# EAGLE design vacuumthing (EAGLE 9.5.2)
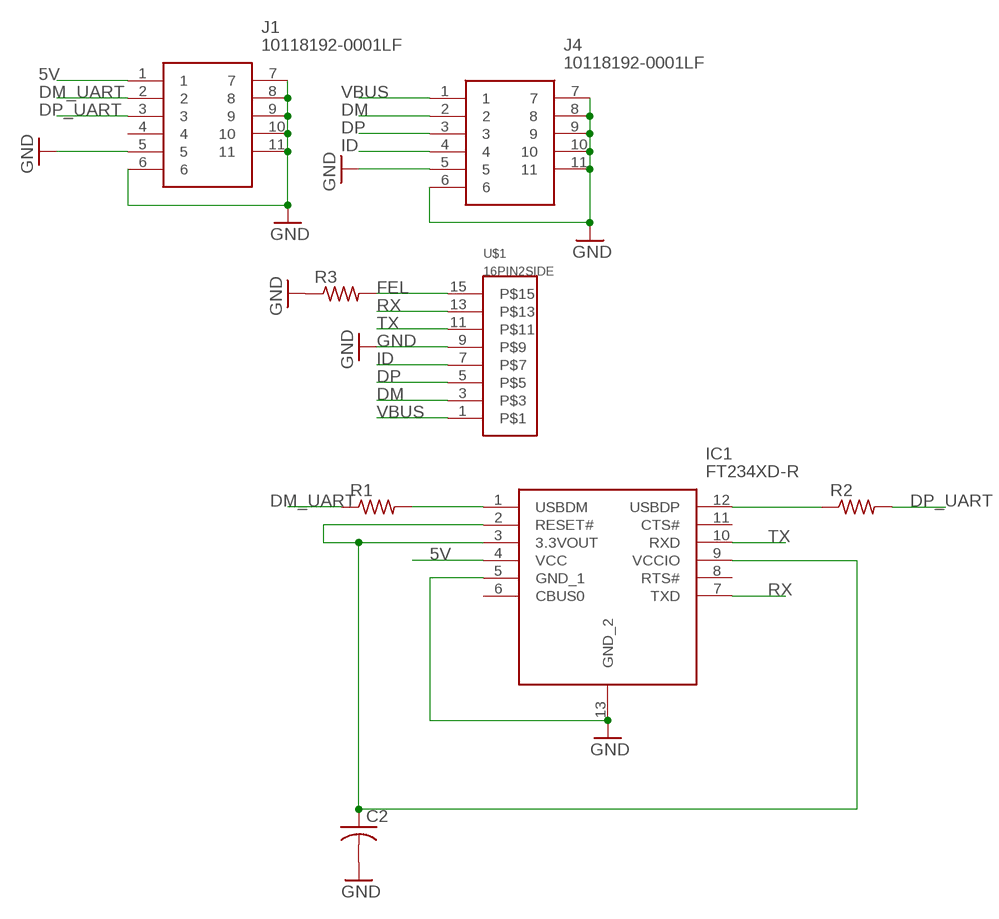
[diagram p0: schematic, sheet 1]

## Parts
C2  C-USC0402K  [C0402K]
IC1  FT234XD-R  [SON45P300X300X75-13N]
J1  10118192-0001LF  [101181920001LF]
J4  10118192-0001LF  [101181920001LF]
R1  R-US_R0402  [R0402]
R2  R-US_R0402  [R0402]
R3  R-US_R0603  [R0603]
U$1  16PIN2SIDE  [16PIN2SIDE]

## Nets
5V: IC1.4(VCC) J1.1
DM: J4.2 U$1.3
DM_UART: J1.2 R1.1
DP: J4.3 U$1.5
DP_UART: J1.3 R2.2
FEL: R3.2 U$1.15
GND: C2.2 IC1.5(GND_1) IC1.13(GND_2) J1.5 J1.6 J1.7 J1.8 J1.9 J1.10 J1.11 J4.5 J4.6 J4.7 J4.8 J4.9 J4.10 J4.11 R3.1 U$1.9
ID: J4.4 U$1.7
N$2: C2.1 IC1.2(RESET#) IC1.3(3.3VOUT) IC1.9(VCCIO)
N$4: IC1.1(USBDM) R1.2
N$7: IC1.12(USBDP) R2.1
RX: IC1.7(TXD) U$1.13
TX: IC1.10(RXD) U$1.11
VBUS: J4.1 U$1.1
Unconnected: IC1.6(CBUS0) IC1.8(RTS#) IC1.11(CTS#) J1.4

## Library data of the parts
C2 = rcl:C-US: CAPACITOR, American symbol; SPICEPREFIX: C
IC1 = SamacSys_Parts:FT234XD-R: USB/UART IC, w/USB Charge Detection FTDI Chip FT234XD-R, USB Controller, 3MBd, USB 1.1, USB 2.0, 5 V, 12-Pin DFN Source: Datasheet; ARROW_PART_NUMBER: FT234XD-R; ARROW_PRICE-STOCK: https://www.arrow.com/en/products/ft234xd-r/ftdi-chip; DESCRIPTION: USB/UART IC, w/USB Charge Detection FTDI Chip FT234XD-R, USB Controller, 3MBd, USB 1.1, USB 2.0, 5 V, 12-Pin DFN; HEIGHT: 0.75mm; MANUFACTURER_NAME: FTDI Chip; MANUFACTURER_PART_NUMBER: FT234XD-R; MOUSER_PART_NUMBER: 895-FT234XD-R; MOUSER_PRICE-STOCK: https://www.mouser.co.uk/ProductDetail/FTDI/FT234XD-R?qs=NVftvxkm2tjipk322Ah1HQ%3D%3D
J1 J4 = SamacSys_Parts:10118192-0001LF: USB Connectors 5P MICRO USB TYPE B RECEPTACLE Source: Datasheet; ARROW_PART_NUMBER: 10118192-0001LF; ARROW_PRICE-STOCK: https://www.arrow.com/en/products/10118192-0001lf/amphenol-fci; DESCRIPTION: USB Connectors 5P MICRO USB TYPE B RECEPTACLE; HEIGHT: 2.8mm; MANUFACTURER_NAME: Amphenol; MANUFACTURER_PART_NUMBER: 10118192-0001LF; MOUSER_PART_NUMBER: 649-10118192-0001LF; MOUSER_PRICE-STOCK: https://www.mouser.co.uk/ProductDetail/Amphenol-FCI/10118192-0001LF/?qs=Ywefl8B65e5bHFoQtIudZg%3D%3D
R1-R3 = rcl:R-US_: RESISTOR, American symbol; SPICEPREFIX: R
U$1 = 16pin2.0:16PIN2SIDE

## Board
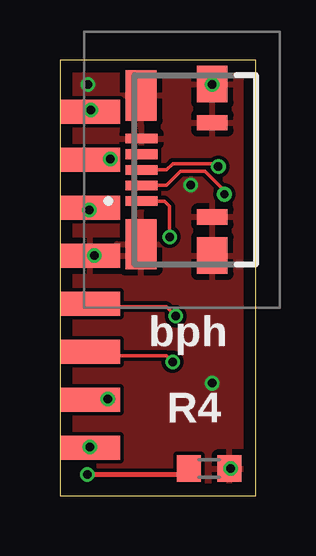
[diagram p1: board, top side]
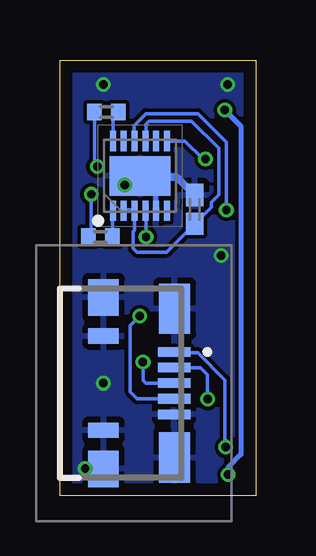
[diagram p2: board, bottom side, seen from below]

Size 8.17 x 18.16 mm. Coordinates in mm from the lower left corner, seen from the top.
Outline: 0,0 8.17,0 8.17,18.16 0,18.16 0,0
Copper layers (1*16): Top 0.035mm / dielectric 1.5mm / Bottom 0.035mm
Design rules "default *": minimum track width 6mil, minimum drill 0.35mm, track to track 6mil, track to pad 6mil, pad to pad 6mil, via to via 6mil, smd to smd 6mil, copper to edge 20mil, drill to drill 6mil, minimum pad ring 10mil, minimum via ring 0.13mm, stop-mask expansion 0mil, vias tented up to drill 30mil, thermal gap 10mil

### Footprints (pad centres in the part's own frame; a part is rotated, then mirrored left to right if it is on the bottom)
C0402K = smd 0.925 x 0.74: 1 -0.6,0; 2 0.6,0
SON45P300X300X75-13N = smd 0.85 x 0.25: 1 -1.45,1.125; 2 -1.45,0.675; 3 -1.45,0.225; 4 -1.45,-0.225; 5 -1.45,-0.675; 6 -1.45,-1.125; 7 1.45,-1.125; 8 1.45,-0.675; 9 1.45,-0.225; 10 1.45,0.225; 11 1.45,0.675; 12 1.45,1.125 | smd 1.65 x 2.55: 13 0,0
101181920001LF = smd 0.4 x 1.35: 1 -1.3,1.682; 2 -0.65,1.682; 3 0,1.682; 4 0.65,1.682; 5 1.3,1.682 | smd 2.1 x 1.295: 6 -3.1,1.702; 7 3.1,1.702 | smd 0.635 x 1.27: 8 -1.962,-1.27; 9 1.962,-1.27 | smd 1.524 x 1.27: 10 -3.571,-1.27; 11 3.571,-1.27
R0402 = smd 0.6 x 0.7: 1 -0.5,0; 2 0.5,0
R0603 = smd 1 x 1.1: 1 -0.85,0; 2 0.85,0
16PIN2SIDE = smd 2.5 x 1: 1 0,0; 3 0,2; 5 0,4; 7 0,6; 9 0,8; 11 0,10; 13 0,12; 15 0,14

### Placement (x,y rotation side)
C2  2.55,11.94 90 bottom
IC1  4.83,13.33 90 bottom
J1  5.09,13.59 90 top
J4  5.09,4.7 270 bottom
R1  6.49,10.79 0 bottom
R2  6.23,16 180 bottom
R3  6.23,1.14 180 top
U$1  1.25,2.02 0 top

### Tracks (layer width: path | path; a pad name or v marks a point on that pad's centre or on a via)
5V  (via drill 0.35)
  Top 0.152: J1.1 4.36,12.29 4.58,12.06 v4.58,10.79
  Bottom 0.152: v4.58,10.79 4.58,11.86 IC1.4
DM  (via drill 0.35)
  Top 0.152: U$1.3 1.87,4.02 v2.01,4.04
  Bottom 0.152: J4.2 2.31,5.35 2.01,5.05 v2.01,4.04
DM_UART  (via drill 0.35)
  Top 0.152: v6.87,12.57 6.87,12.71 6.05,13.53 5.03,13.53 4.44,12.94 J1.2
  Bottom 0.152: R1.1 6.87,10.91 v6.87,12.57
DP  (via drill 0.35)
  Top 0.152: v4.71,5.59 4.45,5.84 1.54,5.84 U$1.5
  Bottom 0.152: J4.3 4.58,4.7 4.71,4.83 v4.71,5.59
DP_UART  (via drill 0.35)
  Top 0.152: v6.61,13.72 6.49,13.85 4.71,13.85 4.45,13.59 J1.3
  Bottom 0.152: R2.2 6.73,13.84 v6.61,13.72
FEL  (via drill 0.35)
  Top 0.203: R3.2 5.13,0.89 v1.15,0.89 | v1.29,16.08 1.47,15.92 U$1.15
  Bottom 0.203: v1.15,0.89 1.15,1.19 0.61,1.73 0.61,15.4 v1.29,16.08
GND  (via drill 0.35)
  Bottom 0.203: 5.51,12.66 4.9,13.27 IC1.13 | IC1.5 4.16,12.72 4.71,13.27
  Bottom 0.305: C2.2 3.28,13.27 4.71,13.27 4.9,13.27
  other vias: 1.44,10.02 1.17,17.14 6.36,17.14 7.12,1.14 6.36,4.7 5.46,12.96
  pour Bottom: -1.77,19.94 -1.77,-1.65 9.66,-1.65 9.66,19.94
  pour Top: -1.77,19.94 -1.77,-1.65 9.66,-1.65 9.66,19.94
ID  (via drill 0.35)
  Top 0.152: v4.83,7.49 4.45,7.87 1.54,7.87 U$1.7
  Bottom 0.152: J4.4 4.95,4.05 5.24,4.34 5.24,7.09 v4.83,7.49
N$2
  Bottom 0.152: IC1.9 4.58,14.81 4.58,15.49 4.45,15.62 2.67,15.62 1.53,14.48 1.53,12.55 1.85,12.24 1.85,12.04 C2.1 3.73,10.16 4.96,10.16 5.11,10.31 5.11,11.02 5.06,11.07 IC1.3
  Bottom 0.203: IC1.3 IC1.2
N$4
  Bottom 0.152: IC1.1 5.99,11.86 R1.2
N$7
  Bottom 0.152: R2.1 5.96,15.77 IC1.12
RX  (via drill 0.35)
  Top 0.152: v2.1,14.05 1.93,13.88 U$1.13
  Bottom 0.152: v2.1,14.05 2.21,14.05 2.95,14.79 IC1.7
TX  (via drill 0.35)
  Top 0.152: U$1.11 1.25,11.95 v1.22,11.92
  Bottom 0.152: v1.22,11.92 1.22,12.22 1.23,12.22 1.23,14.74 2.41,15.93 4.58,15.93 5.09,15.41 5.09,14.82 IC1.10
VBUS  (via drill 0.35)
  Top 0.152: U$1.1 1.27,2.02 v1.25,2.04
  Bottom 0.152: J4.1 3.38,5.97 2.42,5.97 1.28,4.83 1.28,2.06 v1.25,2.04

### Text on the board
tNames: bph | R4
